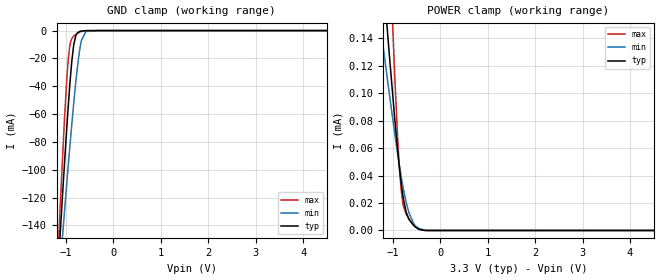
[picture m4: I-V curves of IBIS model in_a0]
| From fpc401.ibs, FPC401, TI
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|   in_a0 Model
[Model]   in_a0
Model_type   Input
Vinl = 0.8
Vinh = 2
|   typ   min   max
C_comp   1.080e-12   1.078e-12   1.087e-12
| Where nom  PVT is Nominal Process, 3.3V, 27C
|   Fast PVT is Strong Process,  3.6V, -40C
|   Slow PVT is Weak Process,   3V, 125C
[Voltage Range]   3.3   3   3.6
|Junction Temperature
[Temperature Range]   27   125   -40
[Power Clamp Reference]   3.3   3   3.6
[GND Clamp Reference]   0   0   0
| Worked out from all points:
|   GND clamp passes 1 mA (typ) near -0.73 V on its own axis
[GND Clamp]
|   Voltage   I(typ)   I(min)   I(max)
-3.3V     -1.497A    -1.178A    -1.889A
-1.197V   -189.1mA   -201.8mA   -181.8mA
-1.115V   -141.5mA   -165.7mA   -120.7mA
-1.076V   -119.5mA   -148.9mA   -92.97mA
-985.2mV  -70.57mA   -110.5mA   -35.84mA
-924mV    -40.87mA   -85.43mA   -11.9mA
-838.2mV  -10.51mA   -52.44mA   -3.986mA
-720mV    -732.9uA   -15.76mA   -1.234mA
-672mV    -304.1uA   -6.775mA   -613.8uA
-582mV    -52.5uA    -738.5uA   -104.3uA
-330mV    -89.36nA   -744.8nA   -56.52nA
6.6V      0A         0A         0A
[POWER Clamp]
|   Voltage   I(typ)   I(min)   I(max)
-3.3V     1.156mA    727.3uA    2.344mA
-1.251V   204.1uA    146.3uA    368.3uA
-1.2V     181.9uA    132.7uA    321.6uA
-1.082V   131.3uA    101.5uA    215.6uA
-1.061V   122.2uA    95.94uA    196.6uA
-960mV    81.27uA    70.45uA    112.1uA
-906mV    60.85uA    57.44uA    72.14uA
-862.8mV  45.91uA    47.53uA    45.99uA
-792mV    26uA       32.73uA    20.37uA
-663.3mV  8.201uA    13.21uA    8.723uA
-456mV    938.5nA    1.48uA     846.4nA
6.6V      0A         0A         0A
